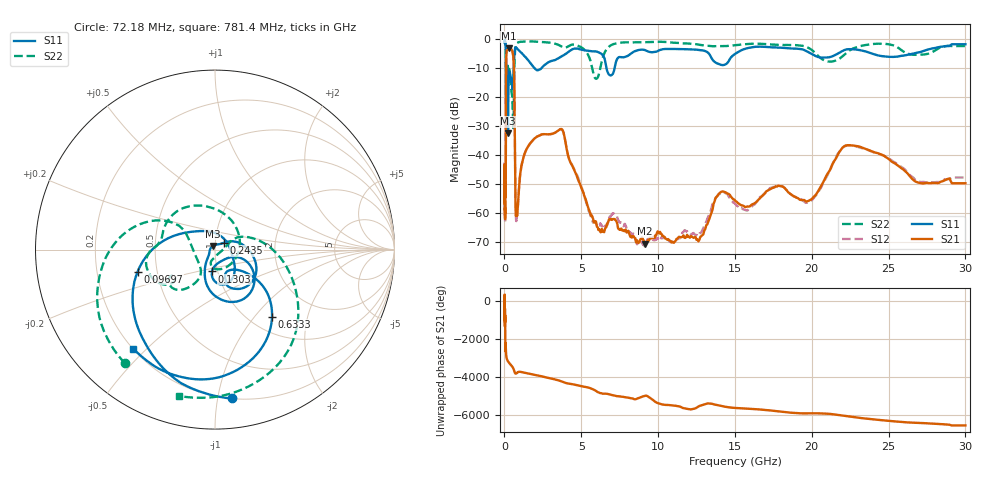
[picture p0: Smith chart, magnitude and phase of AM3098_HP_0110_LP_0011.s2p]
! Date/Time: Thu, Feb 28, 2019 8:37 AM
! Network Analyzer: Agilent Technologies E8364B Rev: A.07.50.67
! Sweep from 0.010 to 30.000 GHz, 1601 Points, Sweep Type: LOG
! Power Supply: 5.022 V, 0.002 A
# Hz S DB R 50
!freq MagS11 AngS11 MagS21 AngS21 MagS12 AngS12 MagS22 AngS22
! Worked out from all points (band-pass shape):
!   1601 points, 10 MHz to 30 GHz, reference 50 ohm
!   highest |S21| = -3.07 dB at 269.1 MHz (marker M1); lowest = -70.4 dB at 9.164 GHz (marker M2)
!   |S21| within 3 dB of the highest: 117.4 MHz to 577 MHz (459.7 MHz wide, 132 % of centre)
!   lowest |S11| = -32.4 dB at 231.6 MHz (marker M3), VSWR 1.05, Z = 48.6 + j1.93 ohm
!   |S11| at or under -10 dB: 174.7 MHz to 598.5 MHz (423.8 MHz wide, 110 % of centre); 1.977 GHz to 2.396 GHz (419.2 MHz wide, 19.2 % of centre); 6.644 GHz to 7.165 GHz (521.2 MHz wide, 7.55 % of centre)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
!   |S22| runs from -30.6 to -0.5 dB; largest |S21 - S12| = 0.013
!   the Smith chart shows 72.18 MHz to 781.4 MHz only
!   S11 on the Smith chart (normalised r, x): 72.18 MHz: 0.20, -1.10; 96.97 MHz: 0.39, -0.12; 130.3 MHz: 0.94, -0.23; 243.5 MHz: 1.10, +0.08; 633.3 MHz: 1.25, -1.24; 781.4 MHz: 0.20, -0.46
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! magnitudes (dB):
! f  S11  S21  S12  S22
! 10 MHz  -0.3  -43.8  -43.4  -0.5
! 38.04 MHz  -0.5  -60.7  -60.5  -0.8
! 72.18 MHz  -1.6  -52.2  -52.4  -1.9
! 84.29 MHz  -2.7  -50.1  -50.3  -2.9
! 96.97 MHz  -7.0  -24.7  -24.8  -8.0
! 130.3 MHz  -18.2  -4.7  -4.7  -10.4
! 144.7 MHz  -18.5  -3.9  -3.9  -11.2
! 185.8 MHz  -11.0  -3.6  -3.6  -8.1
! 231.6 MHz  -32.4  -3.2  -3.1  -9.8
! 243.5 MHz  -24.2  -3.1  -3.1  -10.1
! 269.1 MHz  -15.2  -3.1  -3.0  -10.3
! 550.5 MHz  -15.9  -5.0  -4.9  -27.1
! 633.3 MHz  -6.2  -13.6  -13.5  -12.1
! 721.3 MHz  -2.7  -57.1  -56.8  -2.3
! 781.4 MHz  -2.9  -60.1  -62.4  -1.5
! 2.084 GHz  -10.5  -33.7  -33.6  -0.7
! 3.723 GHz  -5.8  -30.9  -31.0  -2.4
! 7.926 GHz  -5.9  -66.5  -64.7  -1.0
! 9.164 GHz  -3.7  -70.4  -71.1  -0.9
! 19.7 GHz  -4.2  -55.9  -56.4  -2.7
! 22.67 GHz  -3.4  -36.6  -36.7  -3.2
! 30 GHz  -1.6  -49.6  -47.6  -2.3
